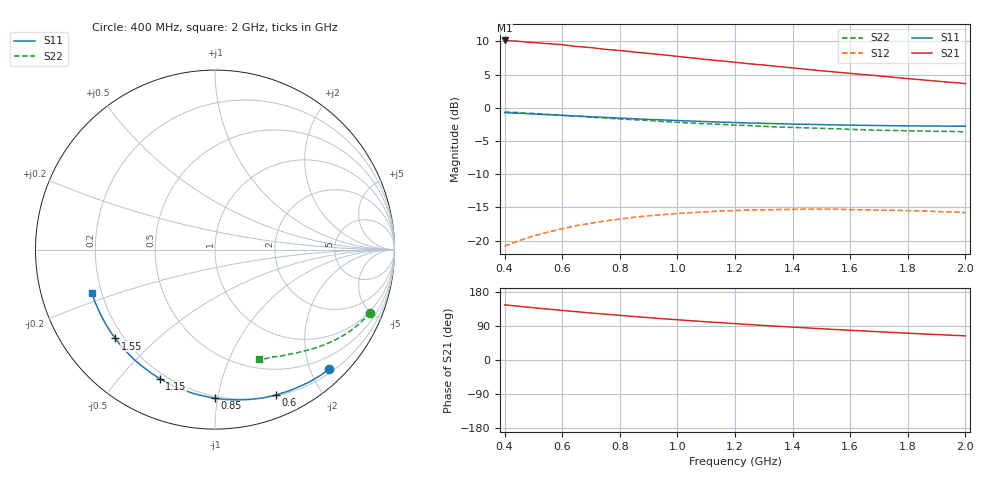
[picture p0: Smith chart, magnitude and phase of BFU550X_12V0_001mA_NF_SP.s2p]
! Filename:  P:\Prog\Test\Noise\ATS_data\Testdata_Net\BFU550X no attenuator noise\BFU550X_APG2013_44_C05_12p0V_001mA_NF_CM01_D.sf
! Date/Time: Fri 26/Jul/2013 14:37:13
! BFU550X_APG2013_44_C05_12p0V_1to10mA_NF_CM01_Bias1_R.sf
! Noise Parameter Data File
! BFU550X_APG2013_44_C05_12p0V_1to10mA_NF_CM01
! Date/time: Thu Jul 25 09:36:35 2013
! freq range =  0.4000 to  2.0000 GHz, 37 points
! bias range =  0.9950 to  9.9950 mA, 5 points
! bias supplies used: 1 1 0 0 0 0
! VAR bias_mode= 1  ! Specify V_out, I_out
! VAR bias_var = 1  ! Bias variable = I_out
! VAR V_out= 12.001000
! VAR I_out= 0.995000
! VAR V_in= 0.771900
! VAR I_in= 0.008400
! Device data file deembeded for feedlines and parallel
! Original file: \BFU550X no attenuator noise\BFU550X_APG2013_44_C05_12p0V_001mA_NF_CM01_R.sf
! Feed-files: PR005V01_100713_Feed1.s2p, PR005V01_100713_Feed2.s2p
! Parallel-file: PR005V01_100713_Par.s2p
# MHz S MA R 50
!  Freq-MHz  S11-mag  S11-arg  S21-mag  S21-arg  S12-mag  S12-arg  S22-mag  S22-arg
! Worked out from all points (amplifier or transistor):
!   37 points, 400 MHz to 2 GHz, reference 50 ohm
!   highest |S21| = 10.2 dB at 400 MHz (marker M1)
!   |S21| within 3 dB of that: start of sweep to 1.132 GHz
!   unconditionally stable (mu >= 1): nowhere
!   at 500 MHz: K = 0.13, MSG = 14.6 dB, |S12| = -19.3 dB
!   at 1.1 GHz: K = 0.27, MSG = 11.5 dB, |S12| = -15.7 dB
!   at 2 GHz: K = 0.48, MSG = 9.7 dB, |S12| = -15.8 dB
!   lowest NFmin = 0.55 dB at 433 MHz
!   S11 on the Smith chart (normalised r, x): 400 MHz: 0.26, -2.30; 600 MHz: 0.21, -1.48; 850 MHz: 0.19, -0.98; 1.15 GHz: 0.17, -0.64; 1.55 GHz: 0.17, -0.37; 2 GHz: 0.16, -0.16
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400  0.9204 -46.5  3.217 145.5  0.0909 60.6  0.9341 -22.1
440  0.9125 -50.9  3.183 142.5  0.09823 58.1  0.9233 -23.9
480  0.9045 -55.0  3.12 139.5  0.105 55.6  0.9105 -25.8
500  0.899 -57.2  3.105 137.9  0.1084 54.3  0.9076 -26.8
550  0.8887 -62.4  3.045 134.3  0.1158 51.2  0.8921 -29.0
600  0.8779 -67.4  2.991 130.8  0.123 48.4  0.8786 -31.1
650  0.8685 -72.1  2.897 127.4  0.1297 45.6  0.866 -33.0
700  0.857 -76.9  2.844 124.0  0.1353 42.9  0.8512 -35.1
750  0.8471 -81.3  2.757 120.9  0.1408 40.4  0.8389 -36.8
800  0.8374 -85.9  2.703 117.8  0.1455 37.9  0.8253 -38.6
850  0.8283 -90.2  2.631 114.7  0.15 35.5  0.8135 -40.2
950  0.8109 -98.4  2.509 108.9  0.157 31.0  0.7889 -43.5
1050  0.7953 -106.0  2.378 103.5  0.1625 26.9  0.7676 -46.4
1150  0.7819 -113.2  2.258 98.5  0.1674 23.1  0.752 -48.9
1200  0.7752 -116.8  2.204 96.0  0.1685 21.2  0.7412 -50.3
1300  0.7643 -123.4  2.102 91.3  0.1706 17.7  0.7259 -52.9
1350  0.7601 -126.5  2.046 89.0  0.1714 16.1  0.7182 -54.0
1500  0.7475 -135.5  1.903 82.5  0.1725 11.4  0.7008 -57.4
1550  0.7438 -138.3  1.86 80.4  0.1724 10.0  0.696 -58.5
1750  0.7336 -148.9  1.698 72.6  0.1694 4.7  0.676 -62.9
1850  0.73 -153.8  1.625 68.9  0.1676 2.3  0.6707 -64.9
2000  0.7275 -160.8  1.525 63.7  0.1626 -0.8  0.66 -68.0
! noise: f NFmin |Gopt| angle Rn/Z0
400  0.6635  0.6617  30.62  0.3266
460  0.6364  0.6261  37.39  0.2844
600  0.7379  0.6329  44.36  0.3685
800  0.7874  0.6317  61.82  0.3002
1000  0.8829  0.6274  76.45  0.2677
1200  0.8964  0.6323  91.65  0.2317
1400  1.08  0.644  104.9  0.2229
1600  0.8911  0.6012  120.7  0.1211
1800  0.9075  0.6273  135.8  0.0836
2000  1.096  0.7151  140.3  0.0907
